(* Logix 5000 AddOnInstructionDefinition export Banner_S100_PD_v5; software revision 33.00 *)

TYPE Banner_S100_4State_v5 :
STRUCT
   PDI_Output_State : SINT;   // 0=Inactive, 1=Active
   PDI_State : SINT;   // 0=State1, 1=State2, 2=State3, 3=State4
   PDO_Job_Input : SINT;   // 0=Off, 1=On
END_STRUCT
END_TYPE

TYPE Banner_S100_Counter_v5 :
STRUCT
   PDI_Button_Group_1_State : SINT;   // 0=Inactive, 1=Active
   PDI_Button_Group_2_State : SINT;   // 0=Inactive, 1=Active
   PDI_Button_Group_3_State : SINT;   // 0=Inactive, 1=Active
   PDI_Button_Group_4_State : SINT;   // 0=Inactive, 1=Active
   PDI_Button_Group_5_State : SINT;   // 0=Inactive, 1=Active
   PDI_Value : REAL;   // Current measure, timer, or counter value.
   PDO_Increment_Count : BOOL;   // Increment the counter on rising edge.
   PDO_Decrement_Count : BOOL;   // Decrement the counter on rising edge.
   Reset_Count : BOOL;   // Reset the count in counter mode
END_STRUCT
END_TYPE

TYPE Banner_S100_Measure_v5 :
STRUCT
   PDI_Button_Group_1_State : SINT;   // 0=Inactive, 1=Active
   PDI_Button_Group_2_State : SINT;   // 0=Inactive, 1=Active
   PDI_Button_Group_3_State : SINT;   // 0=Inactive, 1=Active
   PDI_Button_Group_4_State : SINT;   // 0=Inactive, 1=Active
   PDI_Button_Group_5_State : SINT;   // 0=Inactive, 1=Active
   PDI_Value : REAL;   // Current measure, timer, or counter value.
   PDO_Value : DINT;   // Value describing the level of the device, range determined in Measure Mode Parameter Data.
END_STRUCT
END_TYPE

TYPE Banner_S100_PDIO_v5 :
STRUCT
   Run : Banner_S100_Run_Mode_v5;
   FSFL : Banner_S100_4State_v5;   // Four State Full Logic
   Measure : Banner_S100_Measure_v5;
   Timer : Banner_S100_Timer_v5;
   Counter : Banner_S100_Counter_v5;
   PDI_DT : SINT[6];
   PDO_DT : SINT[32];
END_STRUCT
END_TYPE

TYPE Banner_S100_Run_Mode_v5 :
STRUCT
   PDI_Button_Group_1_State : SINT;   // 0=Inactive, 1=Active
   PDI_Button_Group_2_State : SINT;   // 0=Inactive, 1=Active
   PDI_Button_Group_3_State : SINT;   // 0=Inactive, 1=Active
   PDI_Button_Group_4_State : SINT;   // 0=Inactive, 1=Active
   PDI_Button_Group_5_State : SINT;   // 0=Inactive, 1=Active
   PDO_Animation : SINT;   // 0=Off, 1=Steady, 2=Flash, 3=2 Color Flash, 4=Half/Half Steady, 5= Half/Half Rotate, 6=Chase, 7=Intensity Sweep, 8=2 Color Sweep, 9=Sequence, 10=Wave, 11=Double Wave, 12=2 Color Quadrant, 13= 4 Color Quadrant
   PDO_Speed : SINT;   // 0=Slow, 1=Standard, 2=Fast, 3=Custom
   PDO_Pulse_Pattern : SINT;   // 0=Normal, 1=Strobe, 2=Three Pulse, 3=SOS
   PDO_Static_Sequence_Value : INT;   // 0 to 255
   PDO_Sequence_Start_Location : SINT;   // 0=LED1, 1=LED2, 2=LED3, 3=LED4, 4=LED5, 5=LED6, 6=LED7, 7=LED8, 8=LED9, 9=LED10, 10=LED11, 11=LED12, 12=LED13, 13=LED14, 14=LED15, 15=LED16
   PDO_Top_Chevron : SINT;   // 0=Off, 1=On
   PDO_Right_Chevron : SINT;   // 0=Off, 1=On
   PDO_Bottom_Chevron : SINT;   // 0=Off, 1=On
   PDO_Left_Chevron : SINT;   // 0=Off, 1=On
   Color_1 : SINT;   // 0=Off, 1=Green, 2=Red, 3=Orange, 4=Amber, 5=Yellow, 6=Lime Green, 7=Spring Green, 8=Cyan, 9=Sky Blue, 10=Blue, 11=Violet, 12=Magneta, 13=Rose, 14=White, 15=Custom 1
   Color_2 : SINT;   // 0=Off, 1=Green, 2=Red, 3=Orange, 4=Amber, 5=Yellow, 6=Lime Green, 7=Spring Green, 8=Cyan, 9=Sky Blue, 10=Blue, 11=Violet, 12=Magneta, 13=Rose, 14=White, 15=Custom 1
   Color_3 : SINT;   // 0=Off, 1=Green, 2=Red, 3=Orange, 4=Amber, 5=Yellow, 6=Lime Green, 7=Spring Green, 8=Cyan, 9=Sky Blue, 10=Blue, 11=Violet, 12=Magneta, 13=Rose, 14=White, 15=Custom 1
   Color_4 : SINT;   // 0=Off, 1=Green, 2=Red, 3=Orange, 4=Amber, 5=Yellow, 6=Lime Green, 7=Spring Green, 8=Cyan, 9=Sky Blue, 10=Blue, 11=Violet, 12=Magneta, 13=Rose, 14=White, 15=Custom 1
   Direction : SINT;   // 0=CW, 1=CCW
   Haptic_Feedback : SINT;   // 0=Haptic Disabled, 1=Haptic Enabled
   Audible_Type : SINT;   // 0=Off, 1=Pulse, 2=Wobble, 3=Strobe, 4=Whoop, 5=Stacatto, 6=Siren, 7=Continuous 1, 8= Continuous 2, 10=Jingle. 11=Melody 1, 12= Melody 2, 13=Melody 3, 14=Custom
   Line_1_Text : STRING;   // 13 character String
   Line_2_Text : STRING;   // 13 character String
END_STRUCT
END_TYPE

TYPE Banner_S100_Timer_v5 :
STRUCT
   PDI_Button_Group_1_State : SINT;   // 0=Inactive, 1=Active
   PDI_Button_Group_2_State : SINT;   // 0=Inactive, 1=Active
   PDI_Button_Group_3_State : SINT;   // 0=Inactive, 1=Active
   PDI_Button_Group_4_State : SINT;   // 0=Inactive, 1=Active
   PDI_Button_Group_5_State : SINT;   // 0=Inactive, 1=Active
   PDI_Value : REAL;   // Curren measure, timer, or counter value.
   PDO_Run_Timer : BOOL;   // Run the timer in timer mode
   PDO_Reset_Timer : BOOL;   // Reset the timer in timer mode
END_STRUCT
END_TYPE

ADD_ON_INSTRUCTION Banner_S100_PD_v5   (* revision 5.1 *)
// Revision note:
// Updated Run Mode for correct process data output byte order.
VAR_IN_OUT
   PD : Banner_S100_PDIO_v5; {required}
END_VAR
VAR_INPUT
   Operating_Mode : SINT; {required}
   Byte_Swap : BOOL; {required}
END_VAR
VAR
   Temp_Out : SINT[32]; {access None}
   Temp_In : SINT[6]; {access None}
   Temp_DINT : DINT; {access None}
   Temp_Reverse : DINT; {access None}
END_VAR

ROUTINE Logic   (* ladder *)
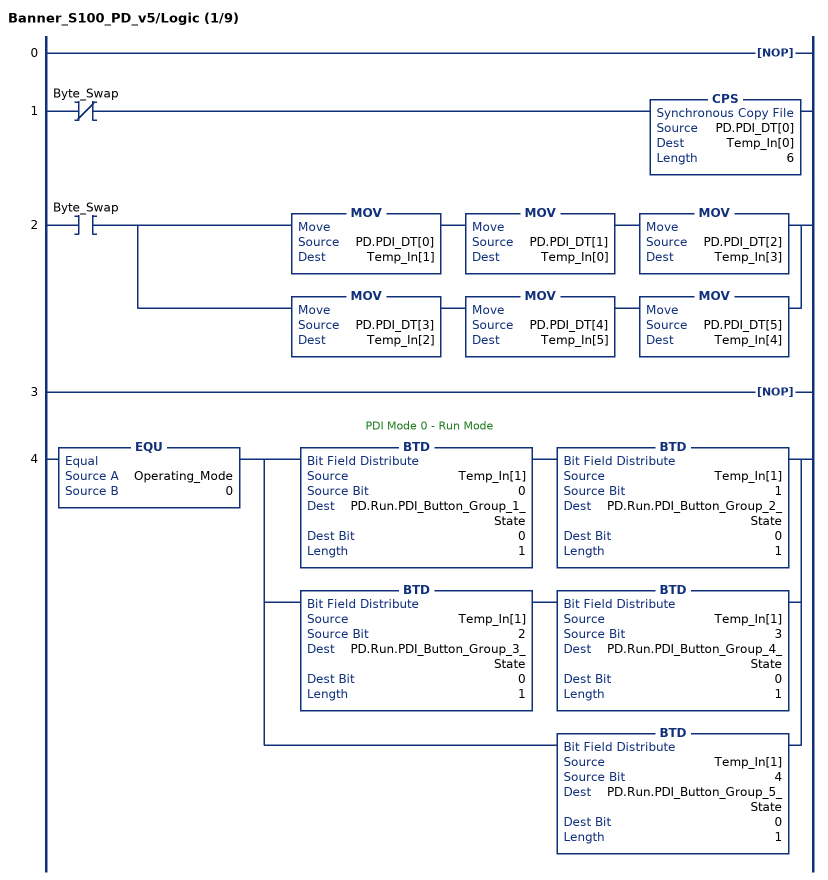
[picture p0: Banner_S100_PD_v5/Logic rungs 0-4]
   0: NOP();
   1: XIO(Byte_Swap)CPS(PD.PDI_DT[0],Temp_In[0],6);
   2: XIC(Byte_Swap)[MOV(PD.PDI_DT[0],Temp_In[1]) MOV(PD.PDI_DT[1],Temp_In[0]) MOV(PD.PDI_DT[2],Temp_In[3]) ,MOV(PD.PDI_DT[3],Temp_In[2]) MOV(PD.PDI_DT[4],Temp_In[5]) MOV(PD.PDI_DT[5],Temp_In[4]) ];
   3: NOP();
   // PDI Mode 0 - Run Mode
   4: EQU(Operating_Mode,0)[BTD(Temp_In[1],0,PD.Run.PDI_Button_Group_1_State,0,1) BTD(Temp_In[1],1,PD.Run.PDI_Button_Group_2_State,0,1) ,BTD(Temp_In[1],2,PD.Run.PDI_Button_Group_3_State,0,1) BTD(Temp_In[1],3,PD.Run.PDI_Button_Group_4_State,0,1) ,BTD(Temp_In[1],4,PD.Run.PDI_Button_Group_5_State,0,1) ];
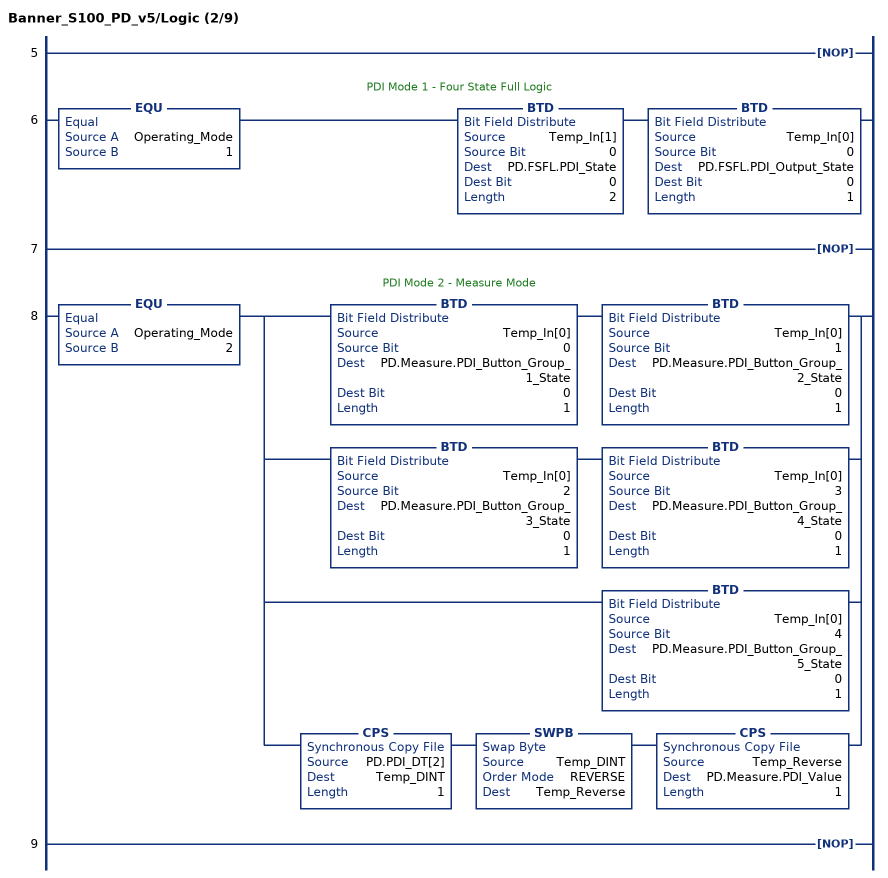
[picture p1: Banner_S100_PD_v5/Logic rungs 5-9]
   5: NOP();
   // PDI Mode 1 - Four State Full Logic
   6: EQU(Operating_Mode,1)BTD(Temp_In[1],0,PD.FSFL.PDI_State,0,2)BTD(Temp_In[0],0,PD.FSFL.PDI_Output_State,0,1);
   7: NOP();
   // PDI Mode 2 - Measure Mode
   8: EQU(Operating_Mode,2)[BTD(Temp_In[0],0,PD.Measure.PDI_Button_Group_1_State,0,1) BTD(Temp_In[0],1,PD.Measure.PDI_Button_Group_2_State,0,1) ,BTD(Temp_In[0],2,PD.Measure.PDI_Button_Group_3_State,0,1) BTD(Temp_In[0],3,PD.Measure.PDI_Button_Group_4_State,0,1) ,BTD(Temp_In[0],4,PD.Measure.PDI_Button_Group_5_State,0,1) ,CPS(PD.PDI_DT[2],Temp_DINT,1) SWPB(Temp_DINT,REVERSE,Temp_Reverse) CPS(Temp_Reverse,PD.Measure.PDI_Value,1) ];
   9: NOP();
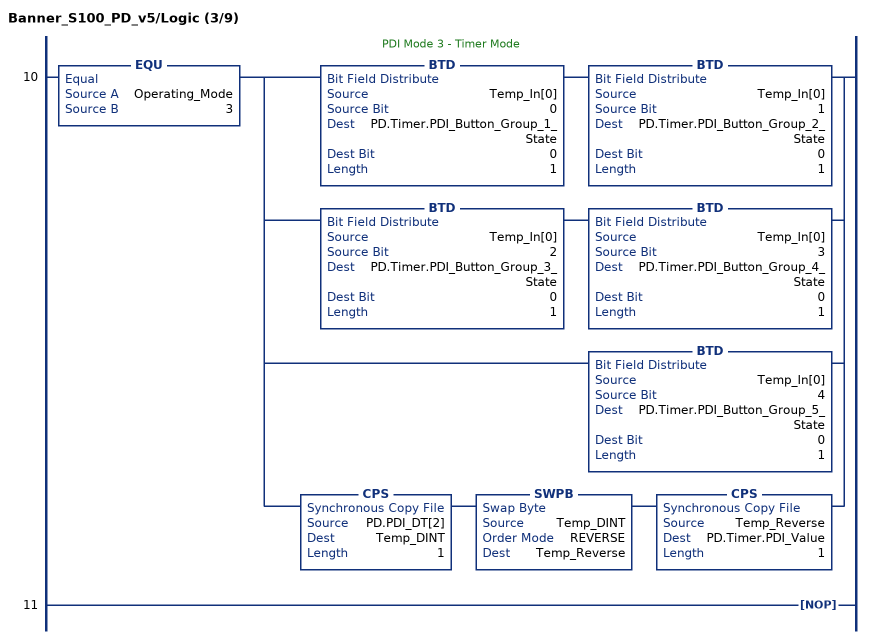
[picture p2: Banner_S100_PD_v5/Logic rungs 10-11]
   // PDI Mode 3 - Timer Mode
   10: EQU(Operating_Mode,3)[BTD(Temp_In[0],0,PD.Timer.PDI_Button_Group_1_State,0,1) BTD(Temp_In[0],1,PD.Timer.PDI_Button_Group_2_State,0,1) ,BTD(Temp_In[0],2,PD.Timer.PDI_Button_Group_3_State,0,1) BTD(Temp_In[0],3,PD.Timer.PDI_Button_Group_4_State,0,1) ,BTD(Temp_In[0],4,PD.Timer.PDI_Button_Group_5_State,0,1) ,CPS(PD.PDI_DT[2],Temp_DINT,1) SWPB(Temp_DINT,REVERSE,Temp_Reverse) CPS(Temp_Reverse,PD.Timer.PDI_Value,1) ];
   11: NOP();
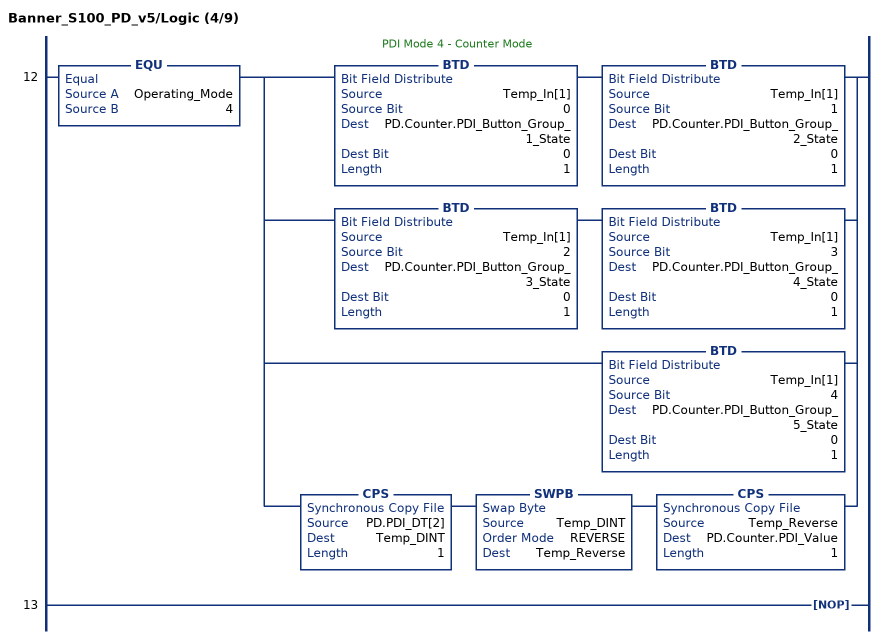
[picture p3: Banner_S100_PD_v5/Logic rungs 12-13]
   // PDI Mode 4 - Counter Mode
   12: EQU(Operating_Mode,4)[BTD(Temp_In[1],0,PD.Counter.PDI_Button_Group_1_State,0,1) BTD(Temp_In[1],1,PD.Counter.PDI_Button_Group_2_State,0,1) ,BTD(Temp_In[1],2,PD.Counter.PDI_Button_Group_3_State,0,1) BTD(Temp_In[1],3,PD.Counter.PDI_Button_Group_4_State,0,1) ,BTD(Temp_In[1],4,PD.Counter.PDI_Button_Group_5_State,0,1) ,CPS(PD.PDI_DT[2],Temp_DINT,1) SWPB(Temp_DINT,REVERSE,Temp_Reverse) CPS(Temp_Reverse,PD.Counter.PDI_Value,1) ];
   13: NOP();
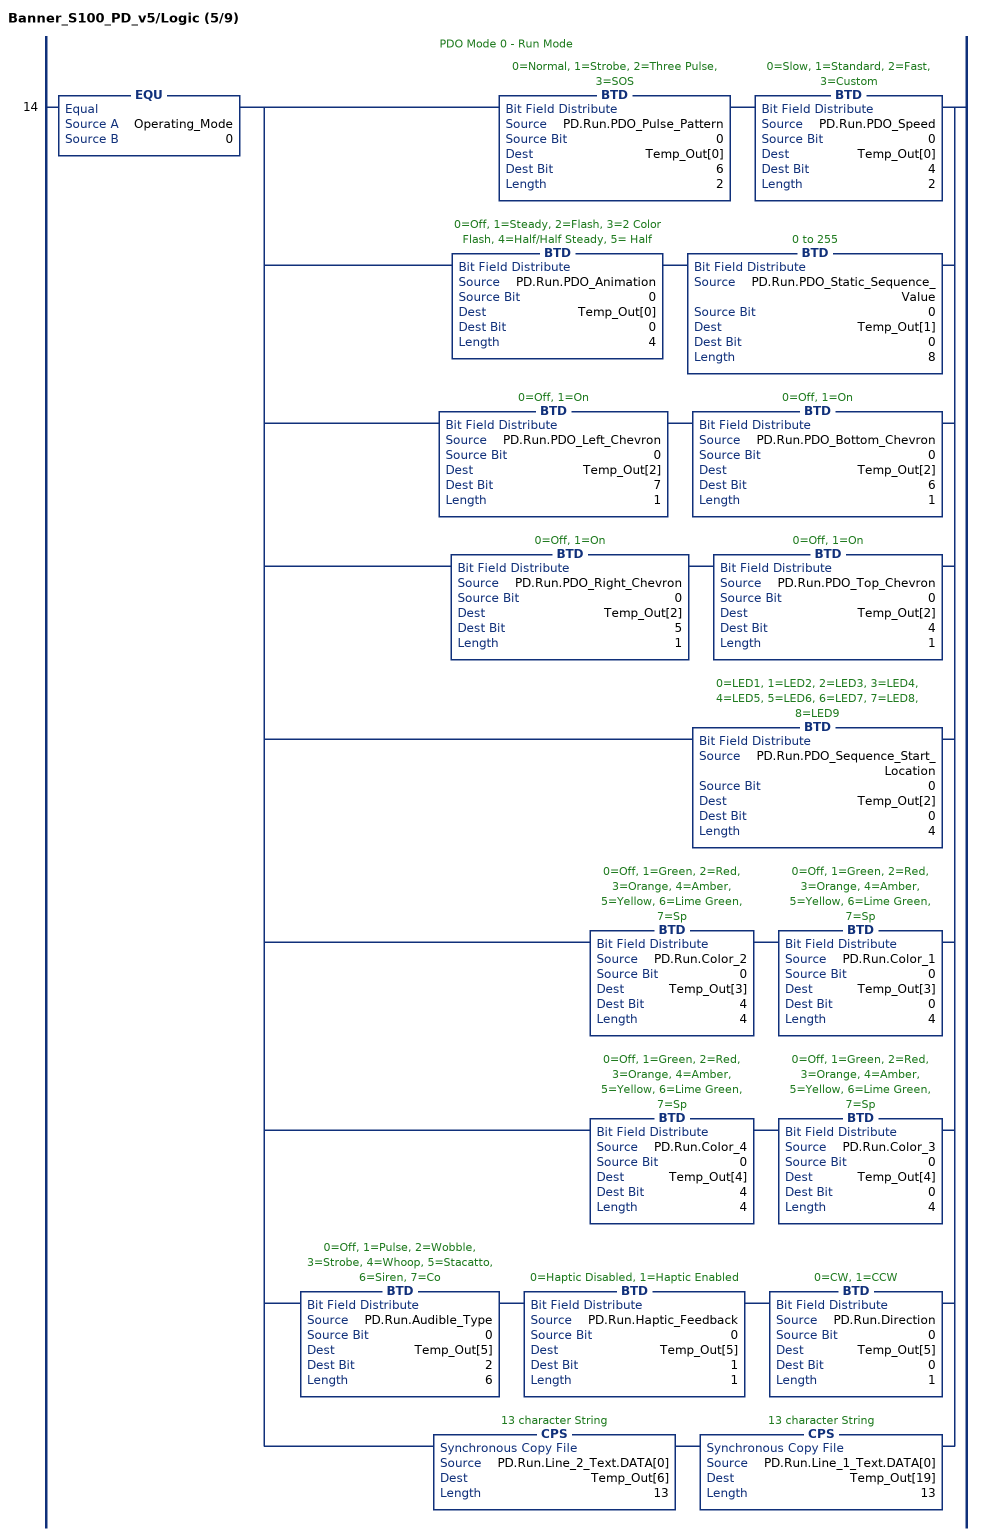
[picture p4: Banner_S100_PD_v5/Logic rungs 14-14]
   // PDO Mode 0 - Run Mode
   14: EQU(Operating_Mode,0)[BTD(PD.Run.PDO_Pulse_Pattern,0,Temp_Out[0],6,2) BTD(PD.Run.PDO_Speed,0,Temp_Out[0],4,2) ,BTD(PD.Run.PDO_Animation,0,Temp_Out[0],0,4) BTD(PD.Run.PDO_Static_Sequence_Value,0,Temp_Out[1],0,8) ,BTD(PD.Run.PDO_Left_Chevron,0,Temp_Out[2],7,1) BTD(PD.Run.PDO_Bottom_Chevron,0,Temp_Out[2],6,1) ,BTD(PD.Run.PDO_Right_Chevron,0,Temp_Out[2],5,1) BTD(PD.Run.PDO_Top_Chevron,0,Temp_Out[2],4,1) ,BTD(PD.Run.PDO_Sequence_Start_Location,0,Temp_Out[2],0,4) ,BTD(PD.Run.Color_2,0,Temp_Out[3],4,4) BTD(PD.Run.Color_1,0,Temp_Out[3],0,4) ,BTD(PD.Run.Color_4,0,Temp_Out[4],4,4) BTD(PD.Run.Color_3,0,Temp_Out[4],0,4) ,BTD(PD.Run.Audible_Type,0,Temp_Out[5],2,6) BTD(PD.Run.Haptic_Feedback,0,Temp_Out[5],1,1) BTD(PD.Run.Direction,0,Temp_Out[5],0,1) ,CPS(PD.Run.Line_2_Text.DATA[0],Temp_Out[6],13) CPS(PD.Run.Line_1_Text.DATA[0],Temp_Out[19],13) ];
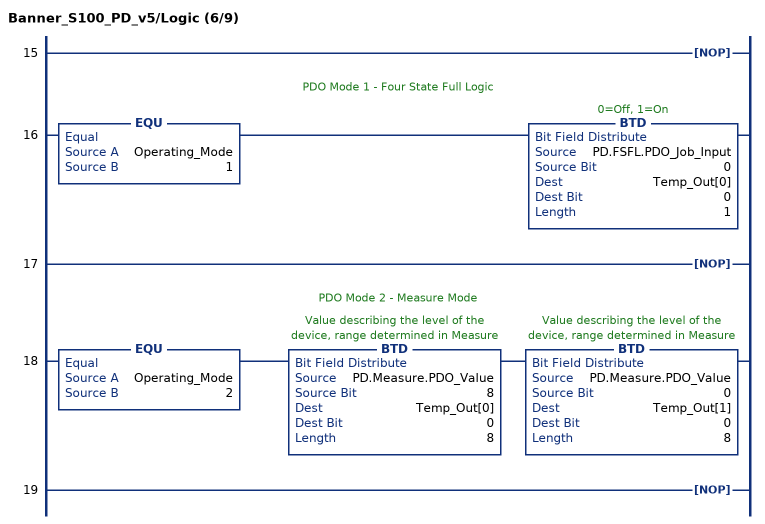
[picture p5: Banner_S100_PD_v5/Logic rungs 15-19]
   15: NOP();
   // PDO Mode 1 - Four State Full Logic
   16: EQU(Operating_Mode,1)BTD(PD.FSFL.PDO_Job_Input,0,Temp_Out[0],0,1);
   17: NOP();
   // PDO Mode 2 - Measure Mode
   18: EQU(Operating_Mode,2)BTD(PD.Measure.PDO_Value,8,Temp_Out[0],0,8)BTD(PD.Measure.PDO_Value,0,Temp_Out[1],0,8);
   19: NOP();
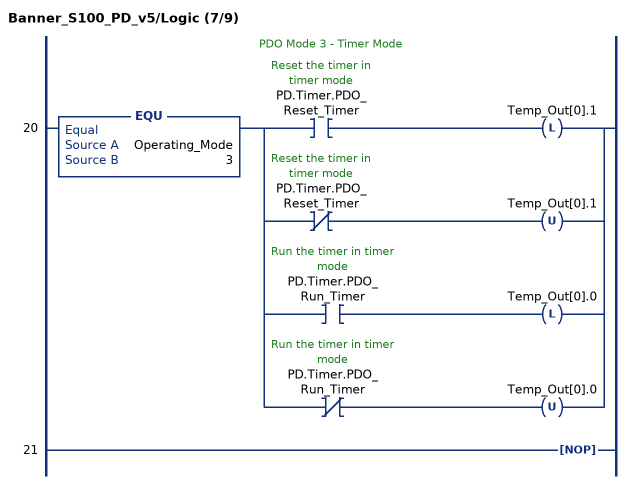
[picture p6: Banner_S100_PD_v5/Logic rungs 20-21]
   // PDO Mode 3 - Timer Mode
   20: EQU(Operating_Mode,3)[XIC(PD.Timer.PDO_Reset_Timer) OTL(Temp_Out[0].1) ,XIO(PD.Timer.PDO_Reset_Timer) OTU(Temp_Out[0].1) ,XIC(PD.Timer.PDO_Run_Timer) OTL(Temp_Out[0].0) ,XIO(PD.Timer.PDO_Run_Timer) OTU(Temp_Out[0].0) ];
   21: NOP();
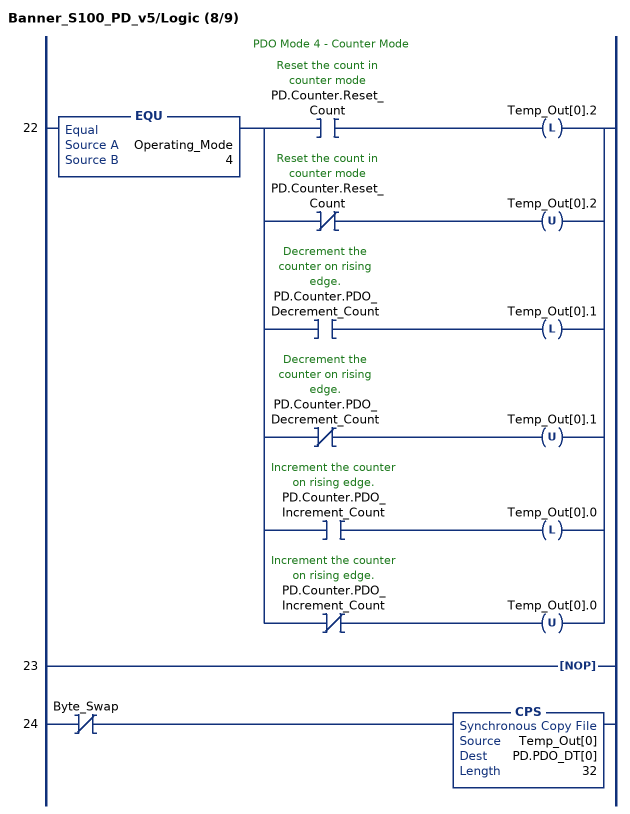
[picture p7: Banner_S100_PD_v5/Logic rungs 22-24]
   // PDO Mode 4 - Counter Mode
   22: EQU(Operating_Mode,4)[XIC(PD.Counter.Reset_Count) OTL(Temp_Out[0].2) ,XIO(PD.Counter.Reset_Count) OTU(Temp_Out[0].2) ,XIC(PD.Counter.PDO_Decrement_Count) OTL(Temp_Out[0].1) ,XIO(PD.Counter.PDO_Decrement_Count) OTU(Temp_Out[0].1) ,XIC(PD.Counter.PDO_Increment_Count) OTL(Temp_Out[0].0) ,XIO(PD.Counter.PDO_Increment_Count) OTU(Temp_Out[0].0) ];
   23: NOP();
   24: XIO(Byte_Swap)CPS(Temp_Out[0],PD.PDO_DT[0],32);
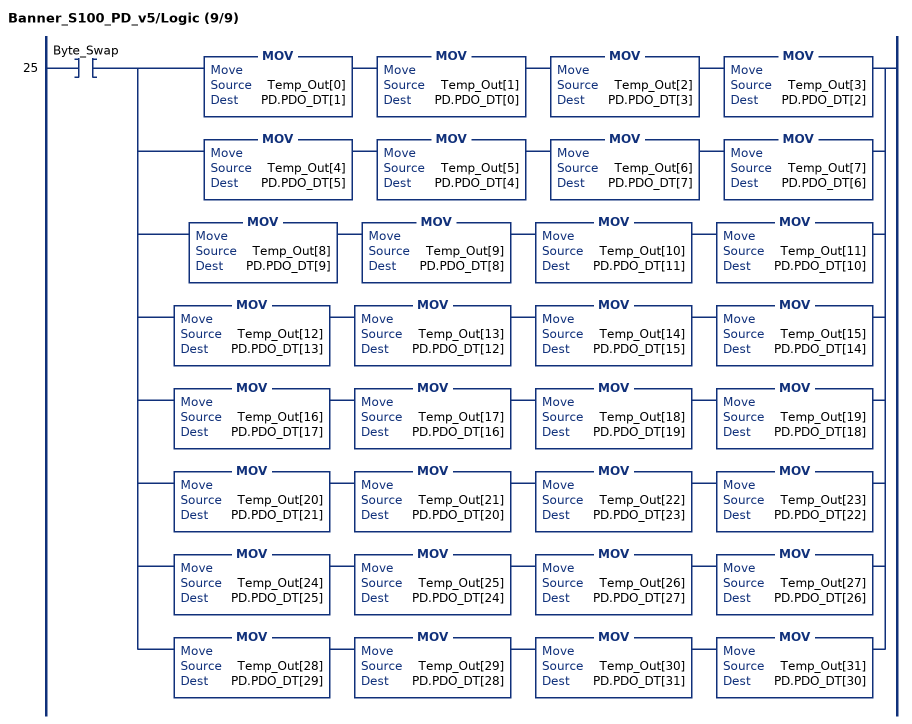
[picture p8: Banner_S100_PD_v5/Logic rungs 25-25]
   25: XIC(Byte_Swap)[MOV(Temp_Out[0],PD.PDO_DT[1]) MOV(Temp_Out[1],PD.PDO_DT[0]) MOV(Temp_Out[2],PD.PDO_DT[3]) MOV(Temp_Out[3],PD.PDO_DT[2]) ,MOV(Temp_Out[4],PD.PDO_DT[5]) MOV(Temp_Out[5],PD.PDO_DT[4]) MOV(Temp_Out[6],PD.PDO_DT[7]) MOV(Temp_Out[7],PD.PDO_DT[6]) ,MOV(Temp_Out[8],PD.PDO_DT[9]) MOV(Temp_Out[9],PD.PDO_DT[8]) MOV(Temp_Out[10],PD.PDO_DT[11]) MOV(Temp_Out[11],PD.PDO_DT[10]) ,MOV(Temp_Out[12],PD.PDO_DT[13]) MOV(Temp_Out[13],PD.PDO_DT[12]) MOV(Temp_Out[14],PD.PDO_DT[15]) MOV(Temp_Out[15],PD.PDO_DT[14]) ,MOV(Temp_Out[16],PD.PDO_DT[17]) MOV(Temp_Out[17],PD.PDO_DT[16]) MOV(Temp_Out[18],PD.PDO_DT[19]) MOV(Temp_Out[19],PD.PDO_DT[18]) ,MOV(Temp_Out[20],PD.PDO_DT[21]) MOV(Temp_Out[21],PD.PDO_DT[20]) MOV(Temp_Out[22],PD.PDO_DT[23]) MOV(Temp_Out[23],PD.PDO_DT[22]) ,MOV(Temp_Out[24],PD.PDO_DT[25]) MOV(Temp_Out[25],PD.PDO_DT[24]) MOV(Temp_Out[26],PD.PDO_DT[27]) MOV(Temp_Out[27],PD.PDO_DT[26]) ,MOV(Temp_Out[28],PD.PDO_DT[29]) MOV(Temp_Out[29],PD.PDO_DT[28]) MOV(Temp_Out[30],PD.PDO_DT[31]) MOV(Temp_Out[31],PD.PDO_DT[30]) ];
END_ROUTINE
END_ADD_ON_INSTRUCTION
